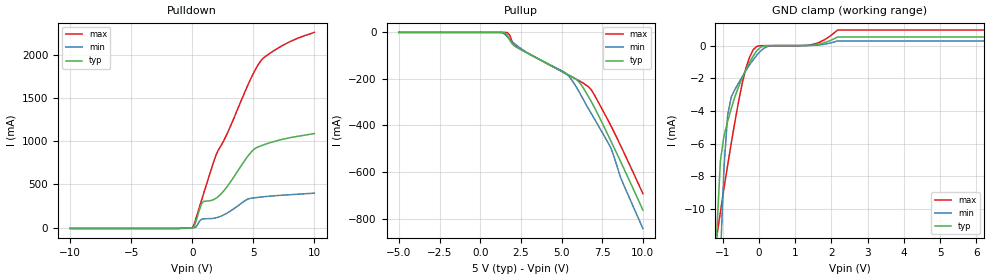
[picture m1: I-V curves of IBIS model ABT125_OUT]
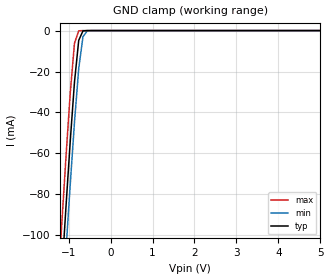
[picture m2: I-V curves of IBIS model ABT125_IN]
|   TEXAS INSTRUMENTS INCORPORATED
|   Advanced Bus Interface Group
|   IBIS Model of SN74ABT125
|   QUADRUPLE BUS BUFFER GATES WITH 3-STATE OUTPUTS
|   14-Pin D,PW,DB,N,NS,RGY Package
[IBIS Ver]   3.2
[Comment char]  |_char
[File Name]   sn74abt125.ibs
[File Rev]   2.1
[Date]   09/13/04
[Source]   File originated at Texas Instruments Incorporated.
[Notes]   The following is a sample IBIS file for the SN74ABT125.
   - This file may be incomplete or may not be fully compliant
   with the IBIS specification. It will be replaced with a
   version that is IBIS Revision 3.2 compliant and is complete
   and accurate. Please email all questions and comments to
   sllibis@ti.com.
   - FILE REV HISTORY
   - 2.1 Release IBIS file on 09/17/04
   - Power clamp data deleted as there is no power-clamp diode.
   - All test data contained in this file are derived from
   hspice(tm) simulations.
[Disclaimer] Property of Texas Instruments Incorporated.  Unauthorized
   reproduction and/or distribution is strictly prohibited.
   This product is protected under copyright law.
   Created 1996, (C) Copyright 1996, Texas Instruments
   Incorporated, All Rights Reserved
   UNLESS THERE IS A SIGNED, WRITTEN AGREEMENT TO THE
   CONTRARY, TEXAS INSTRUMENTS ("TI") IS PROVIDING THE IBIS
   MODELS "AS IS" AND WITHOUT ANY WARRANTY, EXPRESSED OR
   IMPLIED.  TI assumes no liability for:
   1) the accuracy of the IBIS models provided to your
   company;
   2) the proper functioning of these IBIS models in your
   design or for any resulting applications; or
   3) infringement of patents, copyrights or intellectual
   property rights resulting from your use of these IBIS
   models.
   TI provides IBIS Models as a service to our customers.
   You and your company shall not distribute, sell or give
   these models to anyone else without prior written
   permission from TI.
   TI reserves the right to make changes to our products or
   to discontinue any semiconductor product or service
   without notice, and advises our customers to obtain the
   latest version of relevant information to verify, before
   placing orders, that the information being relied on is
   current.
   Please be aware that your receipt and use of the IBIS
   information provided shall serve as acceptance of these
   terms and conditions.  If you do not accept these terms,
   you should return or destroy the IBIS models and any
   other accompanying information immediately
| Component ABT125_D 14-pin D
[Component]   ABT125_D
[Manufacturer]  Texas Instruments Incorporated
[Package]
|   Typ.   Min.   Max.
R_pkg   0.031   0.028   0.034
L_pkg   3.109nH   2.462nH   3.889nH
C_pkg   0.473pF   0.363pF   0.628pF
[Pin]   Signal_name   Model_name   R_pin   L_pin   C_pin
1   1OE_BAR   NC   0.033   3.854nH   0.622pF
2   1A   ABT125_IN   0.032   3.188nH   0.473pF
3   1Y   ABT125_OUT   0.028   2.462nH   0.377pF
4   2OE_BAR   NC   0.031   2.596nH   0.363pF
5   2A   ABT125_IN   0.028   2.521nH   0.372pF
6   2Y   ABT125_OUT   0.034   3.25nH   0.476pF
7   GND   GND   0.034   3.889nH   0.628pF
8   3Y   ABT125_OUT   0.034   3.889nH   0.628pF
9   3A   ABT125_IN   0.034   3.25nH   0.476pF
10   3OE_BAR   NC   0.028   2.521nH   0.372pF
11   4Y   ABT125_OUT   0.031   2.596nH   0.364pF
12   4A   ABT125_IN   0.028   2.462nH   0.377pF
13   4OE_BAR   NC   0.032   3.188nH   0.473pF
14   VCC   POWER   0.033   3.854nH   0.622pF
| Component ABT125_DB 14-pin DB
[Component]   ABT125_DB
[Manufacturer]  Texas Instruments Incorporated
[Package]
|   Typ.   Min.   Max.
R_pkg   0.044   0.041   0.046
L_pkg   3.551nH   3.258nH   3.927nH
C_pkg   0.402pF   0.36pF   0.421pF
[Pin]   Signal_name   Model_name   R_pin   L_pin   C_pin
1   1OE_BAR   NC   0.046   3.927nH   0.408pF
2   1A   ABT125_IN   0.044   3.587nH   0.421pF
3   1Y   ABT125_OUT   0.041   3.289nH   0.398pF
4   2OE_BAR   NC   0.042   3.258nH   0.36pF
5   2A   ABT125_IN   0.041   3.286nH   0.403pF
6   2Y   ABT125_OUT   0.044   3.586nH   0.421pF
7   GND   GND   0.046   3.927nH   0.408pF
8   3Y   ABT125_OUT   0.046   3.927nH   0.408pF
9   3A   ABT125_IN   0.044   3.586nH   0.421pF
10   3OE_BAR   NC   0.041   3.286nH   0.403pF
11   4Y   ABT125_OUT   0.043   3.258nH   0.36pF
12   4A   ABT125_IN   0.041   3.289nH   0.398pF
13   4OE_BAR   NC   0.044   3.587nH   0.421pF
14   VCC   POWER   0.046   3.927nH   0.408pF
| Component ABT125_N 14-pin N
[Component]   ABT125_N
[Manufacturer]  Texas Instruments Incorporated
[Package]
|   Typ.   Min.   Max.
R_pkg   0.045   0.037   0.063
L_pkg   5.407nH   3.922nH   6.942nH
C_pkg   0.389pF   0.205pF   0.604pF
[Pin]  Signal_name   Model_name   R_pin   L_pin   C_pin
1   1OE_BAR   NC   0.063   6.942nH   0.604pF
2   1A   ABT125_IN   0.037   6.2nH   0.406pF
3   1Y   ABT125_OUT   0.042   4.389nH   0.322pF
4   2OE_BAR   NC   0.038   3.922nH   0.205pF
5   2A   ABT125_IN   0.039   4.301nH   0.298pF
6   2Y   ABT125_OUT   0.038   5.329nH   0.356pF
7   GND   GND   0.053   6.51nH   0.544pF
8   3Y   ABT125_OUT   0.053   6.437nH   0.539pF
9   3A   ABT125_IN   0.039   5.352nH   0.347pF
10   3OE_BAR   NC   0.042   4.473nH   0.297pF
11   4Y   ABT125_OUT   0.044   4.326nH   0.225pF
12   4A   ABT125_IN   0.042   4.295nH   0.28pF
13   4OE_BAR   NC   0.042   6.318nH   0.418pF
14   VCC   POWER   0.061   6.9nH   0.603pF
| Component ABT125_PW 14-pin PW
[Component]   ABT125_PW
[Manufacturer]  Texas Instruments Incorporated
[Package]
|   Typ.   Min.   Max.
R_pkg   0.032   0.029   0.035
L_pkg   2.378nH   2.17nH   2.68nH
C_pkg   0.314pF   0.27pF   0.335pF
[Pin]   Signal_name   Model_name   R_pin   L_pin   C_pin
1   1OE_BAR   NC   0.033   2.618nH   0.33pF
2   1A   ABT125_IN   0.031   2.313nH   0.317pF
3   1Y   ABT125_OUT   0.03   2.31nH   0.314pF
4   2OE_BAR   NC   0.031   2.173nH   0.272pF
5   2A   ABT125_IN   0.03   2.204nH   0.309pF
6   2Y   ABT125_OUT   0.032   2.315nH   0.317pF
7   GND   GND   0.035   2.68nH   0.335pF
8   3Y   ABT125_OUT   0.033   2.64nH   0.333pF
9   3A   ABT125_IN   0.034   2.347nH   0.319pF
10   3OE_BAR   NC   0.029   2.277nH   0.313pF
11   4Y   ABT125_OUT   0.031   2.17nH   0.27pF
12   4A   ABT125_IN   0.031   2.244nH   0.311pF
13   4OE_BAR   NC   0.033   2.343nH   0.321pF
14   VCC   POWER   0.035   2.657nH   0.332pF
| Component ABT125_NS 14-pin NS
[Component]   ABT125_NS
[Manufacturer]  Texas Instruments, Inc.
[Package]
|   typ   min   max
R_pkg   4.500e-02   3.900e-02   5.400e-02
L_pkg   3.796e-09   2.561e-09   4.952e-09
C_pkg   5.280e-13   2.880e-13   7.100e-13
[Pin]   signal_name   model_name   R_pin   L_pin   C_pin
1   1OE_BAR   NC   4.700e-02   4.867e-09   7.060e-13
2   1A   ABT125_IN   5.100e-02   4.083e-09   5.920e-13
3   1Y   ABT125_OUT   4.100e-02   2.915e-09   3.760e-13
4   2OE_BAR   NC   3.900e-02   2.561e-09   2.880e-13
5   2A   ABT125_IN   4.100e-02   3.101e-09   4.300e-13
6   2Y   ABT125_OUT   4.700e-02   4.047e-09   5.890e-13
7   GND   GND   5.100e-02   4.909e-09   7.000e-13
8   3Y   ABT125_OUT   4.500e-02   4.784e-09   6.940e-13
9   3A   ABT125_IN   5.400e-02   4.176e-09   5.970e-13
10   3OE_BAR   NC   3.900e-02   3.287e-09   4.490e-13
11   4Y   ABT125_OUT   3.900e-02   2.586e-09   2.940e-13
12   4A   ABT125_IN   4.000e-02   2.802e-09   3.710e-13
13   4OE_BAR   NC   4.900e-02   4.080e-09   5.930e-13
14   VCC   POWER   5.200e-02   4.952e-09   7.100e-13
| Component ABT125_RGY 14-pin RGY
[Component]   ABT125_RGY
[Manufacturer]   Texas Instruments, Inc.
[Package]
|   typ   min   max
R_pkg   2.900e-02   2.300e-02   4.100e-02
L_pkg   7.730e-10   6.570e-10   9.980e-10
C_pkg   1.360e-13   1.150e-13   1.560e-13
[Pin]   signal_name   model_name   R_pin   L_pin   C_pin
1   1OE_BAR   NC   2.700e-02   8.310e-10   1.300e-13
2   1A   ABT125_IN   2.700e-02   8.660e-10   1.350e-13
3   1Y   ABT125_OUT   4.100e-02   9.980e-10   1.560e-13
4   2OE_BAR   NC   3.100e-02   7.670e-10   1.420e-13
5   2A   ABT125_IN   3.100e-02   7.650e-10   1.420e-13
6   2Y   ABT125_OUT   3.100e-02   7.830e-10   1.440e-13
7   GND   GND   3.100e-02   7.810e-10   1.370e-13
8   3Y   ABT125_OUT   2.300e-02   6.570e-10   1.150e-13
9   3A   ABT125_IN   2.300e-02   8.140e-10   1.290e-13
10   3OE_BAR   NC   2.800e-02   7.040e-10   1.290e-13
11   4Y   ABT125_OUT   2.700e-02   6.720e-10   1.360e-13
12   4A   ABT125_IN   2.700e-02   6.960e-10   1.380e-13
13   4OE_BAR   NC   2.700e-02   7.250e-10   1.400e-13
14   VCC   POWER   3.000e-02   7.630e-10   1.360e-13
| Models and submodels in the file (2): ABT125_OUT (3-state), ABT125_IN (Input)
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| Model ABT125__OUT
[Model]   ABT125_OUT
Model_type   3-state
Polarity   Inverting
Enable   Active-Low
|   typ   min   max
C_comp   6.25pF   NA   NA
[Temperature Range]   25   -40   85
[Voltage range]   5.0   4.5   5.5
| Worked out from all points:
|   slope of the pulldown table from 0 to 0.75 V, typ, clamps not added: 2.74 ohm
|   GND clamp passes 1 mA (typ) near -0.25 V on its own axis
[Pullup]
|Voltage   I(typ)   I(min)   I(max)
-5V       6.492nA    6.521nA    5.173nA
1.212V    -4.86uA    -147.7uA   -13.56nA
1.667V    -11.95mA   -19mA      -721.4uA
1.818V    -34.26mA   -30.41mA   -12mA
2.121V    -59.14mA   -49.23mA   -57.87mA
2.879V    -88.71mA   -87.02mA   -87.36mA
5.303V    -178mA     -177.7mA   -179.1mA
6.061V    -211.8mA   -253mA     -207.5mA
6.818V    -296.2mA   -347.8mA   -246.2mA
8.03V     -466.8mA   -496.7mA   -400.8mA
8.636V    -556.5mA   -625.1mA   -487.9mA
10V       -764mA     -843.6mA   -693.3mA
[Pulldown]
|Voltage   I(typ)   I(min)   I(max)
-10V      -5.091mA   -12.04mA   -9.061mA
0V        -2.752mA   -1.654mA   -5.209mA
151.5mV   9.334mA    -1.484mA   38.64mA
757.6mV   274.2mA    96.85mA    316.2mA
909.1mV   304mA      101.8mA    384.9mA
1.97V     342.8mA    114.6mA    848.8mA
2.879V    479.5mA    170.4mA    1.095A
4.697V    852.9mA    337.1mA    1.695A
5.455V    938mA      351.5mA    1.899A
5.909V    962.3mA    358.3mA    1.974A
7.121V    1.014A     373mA      2.088A
10V       1.09A      399.3mA    2.262A
[GND_Clamp]
|Voltage   I(typ)   I(min)   I(max)
-5V       -763mA     -764mA     -762mA
-1.16V    -11.5mA    -20.4mA    -11.7mA
-1.06V    -7.07mA    -13.1mA    -10.2mA
-960mV    -5.52mA    -7.48mA    -8.72mA
-859mV    -4.63mA    -4.24mA    -7.31mA
-758mV    -3.84mA    -3.13mA    -5.94mA
-354mV    -1.47mA    -1.52mA    -1.37mA
-152mV    -623uA     -855uA     -242uA
50.5mV    -95.7uA    -327uA     -3.95uA
1.46V     23.6uA     13.9uA     62.1uA
2.17V     529uA      284uA      955uA
10V       529uA      284uA      955uA
[Ramp]
|Variable   typ   min   max
dV/dt_r   1.695/0.672n   1.392/1.172n   1.911/1.085n
dV/dt_f   2.790/1.938n   2.333/3.951n   3.119/0.994n
| Model ABT125__IN
[Model]   ABT125_IN
Model_type   Input
Polarity   Inverting
Vinl = 0.8V
Vinh = 2.0V
|   typ   min   max
C_comp   2.25pF   NA   NA
[Temperature Range]   25   -40   85
[Voltage Range]   5.0   4.5   5.5
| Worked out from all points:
|   GND clamp passes 1 mA (typ) near -0.67 V on its own axis
[GND_Clamp]
|Voltage   I(typ)   I(min)   I(max)
-5V       -1.471A    -1.489A    -1.45A
-1.263V   -152.8mA   -174.2mA   -128.5mA
-1.162V   -119mA     -140.5mA   -94.61mA
-1.061V   -85.89mA   -107.3mA   -61.57mA
-959.6mV  -54.08mA   -75.14mA   -30.54mA
-858.6mV  -25.15mA   -44.8mA    -6.155mA
-757.6mV  -4.763mA   -18.58mA   -104.1uA
-656.6mV  -173.1uA   -3.018mA   -775.1nA
-555.6mV  -3.889uA   -162.2uA   -5.789nA
5V        1nA        1.004nA    1nA
